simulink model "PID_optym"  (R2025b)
settings: Solver=FixedStepAuto  StartTime=0.0  StopTime=10  FixedStep=0.01  RelTol=1e-3
undefined symbols (not defined in the file): D, I, N, P
libraries: simulink_extras x1, slpidlib x1

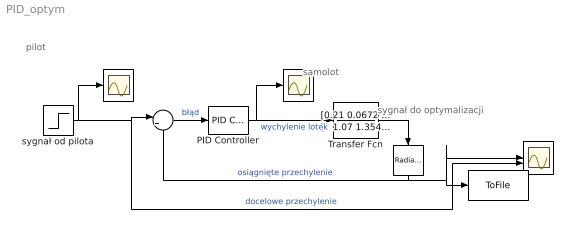
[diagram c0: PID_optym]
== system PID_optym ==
  note: pilot
  note: samolot
  note: sygnał do optymalizacji
  "   " : Scope
  "    " : Scope
  "     " : Scope  NumInputPorts=2
  "      " : simulink_extras/Transformations/Radians to Degrees
  "        " : ToFile  Filename=roll.mat  MatrixName=roll  SaveFormat=Timeseries
  "         " : Sum  Inputs=|+-
  PID Controller : slpidlib/PID Controller  Controller=PID  Form=Parallel  TimeDomain=Continuous-time  UseExternalTs=off  SampleTime=-1  IntegratorMethod=Forward Euler  FilterMethod=Forward Euler  ControllerParametersSource=internal  P=P  I=I  UseKiTs=off  D=D  UseExternalDerivativeSource=off  N=N  UseFilter=on  TunerSelectOption=Transfer Function Based (PID Tuner App)  InitialConditionSource=internal  InitialConditionForIntegrator=0  InitialConditionForFilter=0  DifferentiatorICPrevScaledInput=0  ExternalReset=none  TrackingMode=off  Kt=1  LimitOutput=on  SatLimitsSource=internal  UpperSaturationLimit=20  LowerSaturationLimit=-20  LinearizeAsGain=on  AntiWindupMode=none  Kb=1  LimitIntegrator=off  UpperIntegratorSaturationLimit=inf  LowerIntegratorSaturationLimit=-inf  POutMin=[]  POutMax=[]  IOutMin=[]  IOutMax=[]  DOutMin=[]  DOutMax=[]  NOutMin=[]  NOutMax=[]  SumOutMin=[]  SumOutMax=[]  SaturationOutMin=[]  SaturationOutMax=[]  PParamMin=[]  PParamMax=[]  IParamMin=[]  IParamMax=[]  DParamMin=[]  DParamMax=[]  NParamMin=[]  NParamMax=[]  KbParamMin=[]  KbParamMax=[]  KtParamMin=[]  KtParamMax=[]  KbOutMin=[]  KbOutMax=[]  KtOutMin=[]  KtOutMax=[]  IntegratorOutMin=[]  IntegratorOutMax=[]  FilterOutMin=[]  FilterOutMax=[]  SumI1OutMin=[]  SumI1OutMax=[]  SumI2OutMin=[]  SumI2OutMax=[]  SumI3OutMin=[]  SumI3OutMax=[]  SumI4OutMin=[]  SumI4OutMax=[]  SumDOutMin=[]  SumDOutMax=[]  DifferentiatorOutMin=[]  DifferentiatorOutMax=[]  FilterDiffOutCoefMin=[]  FilterDiffOutCoefMax=[]  ReciprocalOutMin=[]  ReciprocalOutMax=[]  SumDenOutMin=[]  SumDenOutMax=[]  SumNumOutMin=[]  SumNumOutMax=[]  DivideOutMin=[]  DivideOutMax=[]  UdiffTsProdOutMin=[]  UdiffTsProdOutMax=[]  NTsProdOutMin=[]  NTsProdOutMax=[]  UintegralTsProdOutMin=[]  UintegralTsProdOutMax=[]  UngainTsProdOutMin=[]  UngainTsProdOutMax=[]  ClampingZeroOutDataTypeStr=Inherit: Inherit via back propagation  ClampingZeroOutMin=[]  ClampingZeroOutMax=[]  FilterDenConstantOutDataTypeStr=Inherit: Inherit via back propagation  FilterDenConstantOutMin=[]  FilterDenConstantOutMax=[]  PCopyOutDataTypeStr=Inherit: Inherit via back propagation  PCopyOutMin=[]  PCopyOutMax=[]  NCopyOutDataTypeStr=Inherit: Inherit via back propagation  NCopyOutMin=[]  NCopyOutMax=[]  IntegratorContinuousStateAttributes=''  IntegratorStateMustResolveToSignalObject=off  IntegratorRTWStateStorageClass=Auto  FilterContinuousStateAttributes=''  FilterStateMustResolveToSignalObject=off  FilterRTWStateStorageClass=Auto  ParallelPVariant=InternalParameters  IdealPVariant=Disabled  IVariant=InternalParameters  DVariant=InternalParameters  IntegratorVariant=Continuous  SatVariant=Enabled  AWVariant=Passthrough  PCopyVariant=Disabled  TRVariant=Disabled  FdbkBlocksVariant=Forward  IdealPFdbkVariant=Disabled  SatFdbkVariant=Disabled  DerivativeFilterVariant=ContFilter  NVariant=InternalParameters  NCopyVariant=Disabled  FilterICVariant=InternalICsFilter  IntegratorICVariant=InternalICs  ExternalResetVariant=Disabled  TRSumVariant=Passthrough  SumFdbkVariant=Disabled  SumVariant=Sum_PID  TsampFilterVariant=InternalTs  TsampNgainVariant=Passthrough  TsampIntegralVariant=Disabled_SignalSpec  ExternalSaturationOutDataTypeStr=Inherit: Same as second input  DerivativeSourceVariant=ErrorSignal  PreIntVariant=InternalPreInt
  Transfer Fcn : TransferFcn  Numerator=[0.21 0.0672 0.252]  Denominator=[1 1.07 1.3546 1.09344 0.0108]
  sygnał od pilota : Step  Time=0.1  After=30  SampleTime=0
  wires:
  "         "/1 -> PID Controller/1  "błąd"
  sygnał od pilota/1 -> "     "/2, "         "/1, "   "/1  "docelowe przechylenie"
  PID Controller/1 -> Transfer Fcn/1, "    "/1  "wychylenie lotek"
  Transfer Fcn/1 -> "      "/1
  "      "/1 -> "         "/2, "        "/1, "     "/1  "osiągnięte przechylenie"
